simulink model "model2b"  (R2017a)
settings: Solver=ode5  StartTime=0.0  StopTime=100  FixedStep=0.1  RelTol=1e-3
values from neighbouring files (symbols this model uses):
  D = 0    [Mandatory2a.m]    (also in Mandatory2b.m; Mandatory2c.m = 1.25)
  dist_t = 1    [Mandatory2a.m]    (also in Mandatory2b.m = 10; Mandatory2c.m = 10)
  dist_val = 1    [Mandatory2a.m]    (also in Mandatory2b.m; Mandatory2c.m)
  I = 1    [Mandatory2a.m]    (also in Mandatory2b.m = 8.33; Mandatory2c.m = 5)
  K = 5    [Mandatory2a.m]    (also in Mandatory2b.m; Mandatory2c.m)
  P = 2    [Mandatory2a.m]    (also in Mandatory2b.m = 0.7; Mandatory2c.m = 0.84)
  T = 10    [Mandatory2a.m]    (also in Mandatory2b.m; Mandatory2c.m)
  tau = 2    [Mandatory2a.m]    (also in Mandatory2b.m; Mandatory2c.m)
libraries: simulink x2

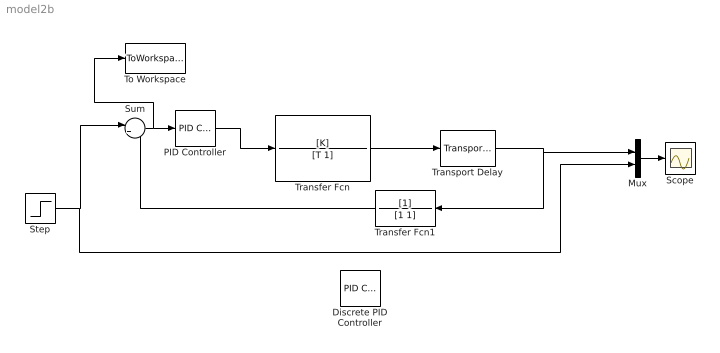
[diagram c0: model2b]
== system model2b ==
  Discrete PID Controller : simulink/Continuous/PID Controller  Controller=PID  TimeDomain=Discrete-time  SampleTime=-1  IntegratorMethod=Forward Euler  FilterMethod=Forward Euler  Form=Parallel  UseFilter=on  ControllerParametersSource=internal  P=1  I=1  D=0  N=100  InitialConditionSource=internal  InitialConditionForIntegrator=0  InitialConditionForFilter=0  ExternalReset=none  LimitOutput=off  UpperSaturationLimit=inf  LowerSaturationLimit=-inf  LinearizeAsGain=off  AntiWindupMode=none  Kb=1  TrackingMode=off  Kt=1  PParamMin=[]  PParamMax=[]  IParamMin=[]  IParamMax=[]  DParamMin=[]  DParamMax=[]  NParamMin=[]  NParamMax=[]  KbParamMin=[]  KbParamMax=[]  KtParamMin=[]  KtParamMax=[]  POutMin=[]  POutMax=[]  IOutMin=[]  IOutMax=[]  DOutMin=[]  DOutMax=[]  NOutMin=[]  NOutMax=[]  KbOutMin=[]  KbOutMax=[]  KtOutMin=[]  KtOutMax=[]  IntegratorOutMin=[]  IntegratorOutMax=[]  FilterOutMin=[]  FilterOutMax=[]  SumOutMin=[]  SumOutMax=[]  SumI1OutMin=[]  SumI1OutMax=[]  SumI2OutMin=[]  SumI2OutMax=[]  SumI3OutMin=[]  SumI3OutMax=[]  SumDOutMin=[]  SumDOutMax=[]  SaturationOutMin=[]  SaturationOutMax=[]  IntegratorContinuousStateAttributes=''  IntegratorStateMustResolveToSignalObject=off  IntegratorRTWStateStorageClass=Auto  FilterContinuousStateAttributes=''  FilterStateMustResolveToSignalObject=off  FilterRTWStateStorageClass=Auto  DifferentiatorICPrevScaledInput=0  DifferentiatorOutMin=[]  DifferentiatorOutMax=[]  InitialConditionSetting=State (most efficient)
  Mux : Mux  Inputs=2
  PID Controller : simulink/Continuous/PID Controller  Controller=PI  TimeDomain=Continuous-time  SampleTime=-1  IntegratorMethod=Forward Euler  FilterMethod=Forward Euler  Form=Parallel  UseFilter=on  ControllerParametersSource=internal  P=P  I=1/I  D=D  N=100  InitialConditionSource=internal  InitialConditionForIntegrator=0  InitialConditionForFilter=0  ExternalReset=none  LimitOutput=off  UpperSaturationLimit=inf  LowerSaturationLimit=-inf  LinearizeAsGain=on  AntiWindupMode=none  Kb=1  TrackingMode=off  Kt=1  PParamMin=[]  PParamMax=[]  IParamMin=[]  IParamMax=[]  DParamMin=[]  DParamMax=[]  NParamMin=[]  NParamMax=[]  KbParamMin=[]  KbParamMax=[]  KtParamMin=[]  KtParamMax=[]  POutMin=[]  POutMax=[]  IOutMin=[]  IOutMax=[]  DOutMin=[]  DOutMax=[]  NOutMin=[]  NOutMax=[]  KbOutMin=[]  KbOutMax=[]  KtOutMin=[]  KtOutMax=[]  IntegratorOutMin=[]  IntegratorOutMax=[]  FilterOutMin=[]  FilterOutMax=[]  SumOutMin=[]  SumOutMax=[]  SumI1OutMin=[]  SumI1OutMax=[]  SumI2OutMin=[]  SumI2OutMax=[]  SumI3OutMin=[]  SumI3OutMax=[]  SumDOutMin=[]  SumDOutMax=[]  SaturationOutMin=[]  SaturationOutMax=[]  IntegratorContinuousStateAttributes=''  IntegratorStateMustResolveToSignalObject=off  IntegratorRTWStateStorageClass=Auto  FilterContinuousStateAttributes=''  FilterStateMustResolveToSignalObject=off  FilterRTWStateStorageClass=Auto  DifferentiatorICPrevScaledInput=0  DifferentiatorOutMin=[]  DifferentiatorOutMax=[]  InitialConditionSetting=State (most efficient)
  Scope : Scope
  Step : Step  Time=dist_t  After=dist_val  SampleTime=0
  Sum : Sum  Inputs=|+-
  To Workspace : ToWorkspace  VariableName=d_error  SampleTime=-1
  Transfer Fcn : TransferFcn  Numerator=[K]  Denominator=[T 1]
  Transfer Fcn1 : TransferFcn  Denominator=[1 1]
  Transport Delay : TransportDelay  DelayTime=tau
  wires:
  Transfer Fcn/1 -> Transport Delay/1
  Step/1 -> Mux/2, Sum/1
  Sum/1 -> To Workspace/1, PID Controller/1
  Mux/1 -> Scope/1
  Transport Delay/1 -> Transfer Fcn1/1, Mux/1
  PID Controller/1 -> Transfer Fcn/1
  Transfer Fcn1/1 -> Sum/2
